(* Logix 5000 AddOnInstructionDefinition export EH_Cerabar_PMP43_IOL; software revision 38.00 *)

TYPE EH_CommAOI_Data :
STRUCT
   Device_Comm_Error : BOOL;
   CommSuccess : BOOL;
   CommFailed : BOOL;
   CommTimeOut : BOOL;
   StateDone : BOOL;
   NewState : BOOL;
   OldState : SINT;
   PortSize : SINT;
   DevicePort : SINT;
   MaxState : SINT;
   State : SINT;
   VendorID : INT;
   DeviceID : DINT;
   CyclicData : INT[16];
   AcyclicData : DINT[8];
   ReplayIndex : INT;
   AOI_Diagnostic : DINT;
   ConnectionStatus : DINT;
   OutputData : INT[16];
END_STRUCT
END_TYPE

ADD_ON_INSTRUCTION EH_Cerabar_PMP43_IOL   (* revision 1.2, vendor Endress+Hauser *)
// Cerabar PMP 43  Rev 1 IO-Link
// Revision note:
// 1.2 Added HeartbeatVerification
// 1.1 Changed the Datatype from Unsigned to Signed
// Add Disconnect check
VAR_IN_OUT
   DataToSend : INT[10]; {required}
   CommAOIBusy : DINT; {required}
   ActiveComPort : DINT; {required}
   DeviceAOISendRequest : DINT; {required}
   CommError : INT; {required}
   DeviceData : EH_CommAOI_Data; {required}
END_VAR
VAR_INPUT
   iSetSimulation : BOOL; {visible}
   iSimulationVariable : INT; {visible}
   iSimulationValue_Pressure : REAL; {visible}
   iSetUnit : BOOL; {visible}
   iUnit : INT; {visible}
   iStart_HeartbeatVerification : BOOL; {visible}
END_VAR
VAR_OUTPUT
   qVendor_ID : DINT; {access Read Only, visible}
   qDevice_ID : DINT; {access Read Only, visible}
   qPressure : REAL; {access None, visible}
   qExtendedDeviceStatus : INT; {access Read Only, visible}
   qUnit : INT; {access Read Only, visible}
   qSSC1_1 : BOOL; {access Read Only, visible}
   qSSC1_2 : BOOL; {access Read Only, visible}
   qVerificationID : INT; {access Read Only, visible}
   qPassed : BOOL; {visible}
   qFailed : BOOL; {visible}
   qAOI_Diagnostic : DINT; {access Read Only, visible}
END_VAR
VAR_IN_OUT
   qAOI_Diagnostic_String : STRING; {required}
END_VAR
VAR_OUTPUT
   qActual_Diagnostics_Code : DINT; {access Read Only, visible}
END_VAR
VAR_IN_OUT
   qActual_Diagnostics_String : STRING; {required}
END_VAR
VAR_OUTPUT
   qLast_Diagnostics_Code : DINT; {visible}
END_VAR
VAR_IN_OUT
   qLast_Diagnostics_String : STRING; {required}
END_VAR
VAR_OUTPUT
   qCommError : DINT; {access None}
   qCommunicationBusy : DINT; {access Read Only, visible}
   qDeviceConnectionError : BOOL; {access Read Only, visible}
END_VAR
VAR
   Temp_DINT : DINT; {access None}
   CMD_Index : INT; {access None}
   CMD_Subindex : INT; {access None}
   CMD_ByteLength : INT; {access None}
   oldCondStatus : INT; {access None}
   oldSetSimulation : SINT; {access None}
   SetSimulation : SINT; {access None}
   SetUnit : SINT; {access None}
   oldSetUnit : SINT; {access None}
   Trigger : BOOL; {access None}
   CMD_Rd : BOOL; {access None}
   CMD_Wr : BOOL; {access None}
   SimulationDINT : DINT; {access None}
   InputByteLength : DINT; {access None}
   AOI_Prio : BOOL; {access None}
   StateMin : DINT; {access None}
   firstTimeDone : BOOL; {access None}
   OldStatus : DINT; {access None}
   CondStatusChanged : BOOL; {access None}
   Calc_ExtendedDeviceStatus : DINT; {access None}
   Totalizer1_DINT : DINT; {access None}
   SimActive : BOOL; {access None}
   CondStatusActive : BOOL; {access None}
   ActiveAOI : BOOL; {access None}
   Skip : BOOL; {access None}
   SimChanged : BOOL; {access None}
   UnitActive : BOOL; {access None}
   UnitChanged : BOOL; {access None}
   DeviceID : DINT; {access None}
   FALSE : BOOL; {access None}
   TRUE : BOOL := 1; {access None}
   temp_string1 : STRING; {access None}
   temp_string2 : STRING; {access None}
   Calc_Pressure : DINT; {access None}
   qPressureTemp : REAL; {access None}
   tempVal : SINT; {access None}
   Start_HeartbeatVerification : SINT; {access None}
   oldStart_HeartbeatVerification : SINT; {access None}
   init : BOOL; {access None}
   SimulationREAL : REAL; {access None}
   StandardTimer : FBD_TIMER; {access None}
   onlyonce : DINT; {access None}
   HeartbeatVerification : BOOL; {access None}
   HeartbeatVerificationActive : BOOL; {access None}
   HeartbeatVerificationChanged : BOOL; {access None}
   b_var : BOOL; {access None}
END_VAR

ROUTINE Logic   (* structured text *)
// Picomag Communication via AL1323
   // =======================================================================
   // Endress+Hauser Digital Solutions
   // ©Copyright (2024) All Rights Reserved
   // =======================================================================
   // Name:                EH_Cerabar_PMP43_IOL
   // Version:             1.2
   // Datum:               11.2025
   // Library:             01.01.00
   // Engineering:         Studio5000 V38.00.00
   // Author:              EH
   // =======================================================================
   
   qAOI_Diagnostic := DeviceData.AOI_Diagnostic;
   qCommunicationBusy := CommAOIBusy;
   DeviceID := 9618689;
   StateMin := 0;
   DeviceData.MaxState := 98;
   
   if DeviceData.DevicePort = 0 or DeviceData.DeviceID <> DeviceID or DeviceData.ConnectionStatus <> 1 then
   
   	qVendor_ID := DeviceData.VendorID;
   	qDevice_ID := DeviceData.DeviceID;
   	qPressure	:= 0;
   	qExtendedDeviceStatus	:= 0;
   	qUnit	:= 0;
   	qSSC1_1	:= FALSE;
   	qSSC1_2	:= FALSE;
   	qActual_Diagnostics_Code	:= 0;
   	qLast_Diagnostics_Code	:= 0;
   	qLast_Diagnostics_String	:= '';
   	qVendor_ID := 0;
   	qPassed := FALSE;
   	qFailed := FALSE;
   	oldCondStatus := 0;
   	CondStatusChanged := FALSE;
   	init := FALSE;
   
   	if DeviceData.DevicePort = 0 then
   
   		qActual_Diagnostics_String	:= 'Device Port is Zero';
   		DeviceData.AOI_Diagnostic.1 := TRUE;
   
   	elsif DeviceData.ConnectionStatus <> 1 then
   
   		qActual_Diagnostics_String	:= 'No Device connected';
   		qDeviceConnectionError := TRUE;
   
   	elsif DeviceData.DeviceID <> DeviceID then
   
   		qActual_Diagnostics_String	:= 'Wrong DeviceID';
   		DeviceData.AOI_Diagnostic.2 := TRUE;
   
   	end_if;
   
   else
   
   	if qActual_Diagnostics_Code = 0  then
   
   		qActual_Diagnostics_String	:= '--------';
   
   	end_if;
   
   	if qLast_Diagnostics_Code = 0 then
   
   		qLast_Diagnostics_String	:= '--------';
   
   	end_if;
   
   	DeviceData.AOI_Diagnostic.1 := FALSE;
   	qDeviceConnectionError := FALSE;
   	DeviceData.AOI_Diagnostic.2  := FALSE;
   
   end_if;
   
   if not DeviceData.AOI_Diagnostic.0
   	and not qDeviceConnectionError
   	and not DeviceData.AOI_Diagnostic.2
   	and DeviceData.DevicePort > 0 or ActiveAOI and qDeviceConnectionError then
   
   	//*********************************
   	//Vendor ID
   	//*********************************
   
   		qVendor_ID := DeviceData.VendorID;
   
   	//*********************************
   	//Device ID
   	//*********************************
   
   		qDevice_ID := DeviceData.DeviceID;
   
   	//*********************************
   	// PMP43
   	//*********************************
   
   		Calc_Pressure				:= 0;
   		Calc_ExtendedDeviceStatus	:= 2;
   
   	//*********************************
   	//Process Data Pressure
   	//*********************************
   
   		Temp_DINT	 := DeviceData.CyclicData[Calc_Pressure+1];
   		Temp_DINT.8	 := DeviceData.CyclicData[Calc_Pressure+1].8;
   		Temp_DINT.9  := DeviceData.CyclicData[Calc_Pressure+1].9;
   		Temp_DINT.10 := DeviceData.CyclicData[Calc_Pressure+1].10;
   		Temp_DINT.11 := DeviceData.CyclicData[Calc_Pressure+1].11;
   		Temp_DINT.12 := DeviceData.CyclicData[Calc_Pressure+1].12;
   		Temp_DINT.13 := DeviceData.CyclicData[Calc_Pressure+1].13;
   		Temp_DINT.14 := DeviceData.CyclicData[Calc_Pressure+1].14;
   		Temp_DINT.15 := DeviceData.CyclicData[Calc_Pressure+1].15;
   		Temp_DINT.16 := DeviceData.CyclicData[Calc_Pressure].0;
   		Temp_DINT.17 := DeviceData.CyclicData[Calc_Pressure].1;
   		Temp_DINT.18 := DeviceData.CyclicData[Calc_Pressure].2;
   		Temp_DINT.19 := DeviceData.CyclicData[Calc_Pressure].3;
   		Temp_DINT.20 := DeviceData.CyclicData[Calc_Pressure].4;
   		Temp_DINT.21 := DeviceData.CyclicData[Calc_Pressure].5;
   		Temp_DINT.22 := DeviceData.CyclicData[Calc_Pressure].6;
   		Temp_DINT.23 := DeviceData.CyclicData[Calc_Pressure].7;
   		Temp_DINT.24 := DeviceData.CyclicData[Calc_Pressure].8;
   		Temp_DINT.25 := DeviceData.CyclicData[Calc_Pressure].9;
   		Temp_DINT.26 := DeviceData.CyclicData[Calc_Pressure].10;
   		Temp_DINT.27 := DeviceData.CyclicData[Calc_Pressure].11;
   		Temp_DINT.28 := DeviceData.CyclicData[Calc_Pressure].12;
   		Temp_DINT.29 := DeviceData.CyclicData[Calc_Pressure].13;
   		Temp_DINT.30 := DeviceData.CyclicData[Calc_Pressure].14;
   		Temp_DINT.31 := DeviceData.CyclicData[Calc_Pressure].15;
   
   		case qUnit of
   
   			//*********************************
   			0: // bar
   			//*********************************
   			COP(Temp_DINT,qPressureTemp,1);
   			qPressure := qPressureTemp / 100000;
   
   			//*********************************
   			6: // psi
   			//*********************************
   			COP(Temp_DINT,qPressureTemp,1);
   			qPressure := qPressureTemp / 6895.7573;
   
   			//*********************************
   			8: // mbar
   			//*********************************
   			COP(Temp_DINT,qPressureTemp,1);
   			qPressure := qPressureTemp / 100;
   
   			//*********************************
   			11: // Pa
   			//*********************************
   			COP(Temp_DINT,qPressure,1);
   
   			//*********************************
   			12: // kPa
   			//*********************************
   			COP(Temp_DINT,qPressureTemp,1);
   			qPressure := qPressureTemp / 1000;
   
   			//*********************************
   			237: // MPA
   			//*********************************
   			COP(Temp_DINT,qPressureTemp,1);
   			qPressure := qPressureTemp / 1000000;
   
   			else // Base unit, Pa
   				COP(Temp_DINT,qPressure,1);
   
   		end_case;
   
   	//*********************************
   	// Extended device Status
   	//*********************************
   
   		qExtendedDeviceStatus.0 := DeviceData.CyclicData[Calc_ExtendedDeviceStatus].8;
   		qExtendedDeviceStatus.1 := DeviceData.CyclicData[Calc_ExtendedDeviceStatus].9;
   		qExtendedDeviceStatus.2 := DeviceData.CyclicData[Calc_ExtendedDeviceStatus].10;
   		qExtendedDeviceStatus.3 := DeviceData.CyclicData[Calc_ExtendedDeviceStatus].11;
   		qExtendedDeviceStatus.4 := DeviceData.CyclicData[Calc_ExtendedDeviceStatus].12;
   		qExtendedDeviceStatus.5 := DeviceData.CyclicData[Calc_ExtendedDeviceStatus].13;
   		qExtendedDeviceStatus.6 := DeviceData.CyclicData[Calc_ExtendedDeviceStatus].14;
   		qExtendedDeviceStatus.7 := DeviceData.CyclicData[Calc_ExtendedDeviceStatus].15;
   
   	//*********************************
   	// Process Parameter SSC
   	//*********************************
   
   		qSSC1_1 := DeviceData.CyclicData[Calc_ExtendedDeviceStatus].0;
   		qSSC1_2 := DeviceData.CyclicData[Calc_ExtendedDeviceStatus].1;
   
   	//*********************************
   	// Checking for Changed Status
   	//*********************************
   
   		SetSimulation.0 := iSetSimulation;
   		SetUnit.0 := iSetUnit;
   		Start_HeartbeatVerification.0 := iStart_HeartbeatVerification;
   
   	if oldCondStatus <> qExtendedDeviceStatus and not CondStatusChanged then
   
   		CondStatusChanged := TRUE;
   		oldCondStatus := qExtendedDeviceStatus;
   
   	end_if;
   
   	if oldSetSimulation <> SetSimulation and not SimChanged then
   
   		if oldSetSimulation < SetSimulation then
   
   			SimChanged := TRUE;
   
   		end_if;
   
   		oldSetSimulation := SetSimulation;
   
   	end_if;
   
   	if oldSetUnit <> SetUnit and not UnitChanged then
   
   		if oldSetUnit < SetUnit then
   
   			UnitChanged := TRUE;
   
   		end_if;
   
   		oldSetUnit := SetUnit;
   
   	end_if;
   
   	if oldStart_HeartbeatVerification <> Start_HeartbeatVerification and not HeartbeatVerificationChanged then
   
   		if oldStart_HeartbeatVerification < Start_HeartbeatVerification then
   
   			HeartbeatVerificationChanged := TRUE;
   
   		end_if;
   
   		oldStart_HeartbeatVerification := Start_HeartbeatVerification;
   
   	end_if;
   
   	if CondStatusChanged
   		and not ActiveAOI
   		and not CondStatusActive
   		and not Skip then
   
   		DeviceAOISendRequest.[DeviceData.DevicePort] := TRUE;
   		CondStatusActive := TRUE;
   		Skip := TRUE;
   
   	elsif SimChanged
   		and not ActiveAOI
   		and not SimActive
   		and not Skip then
   
   		DeviceAOISendRequest.[DeviceData.DevicePort] := TRUE;
   		SimActive := TRUE;
   		Skip := TRUE;
   
   	elsif UnitChanged
   		and not ActiveAOI
   		and not UnitActive
   		and not Skip then
   
   		DeviceAOISendRequest.[DeviceData.DevicePort] := TRUE;
   		UnitActive := TRUE;
   		Skip := TRUE;
   
   	elsif HeartbeatVerificationChanged
   		and not ActiveAOI
   		and not HeartbeatVerificationActive
   		and not Skip then
   
   		DeviceAOISendRequest.[DeviceData.DevicePort] := TRUE;
   		HeartbeatVerificationActive := TRUE;
   		Skip := TRUE;
   
   	end_if;
   
   end_if;
   
   	if ActiveComPort = DeviceData.DevicePort then
   
   		AOI_Prio := TRUE;
   
   	else
   
   		AOI_Prio := FALSE;
   
   	end_if;
   
   	if (SimActive or UnitActive or HeartbeatVerificationActive or CondStatusActive ) and CommAOIBusy = 1  and DeviceData.State = 0 and AOI_Prio and not ActiveAOI then
   
   		ActiveAOI := TRUE;
   		Skip := FALSE;
   
   	end_if;
   
   	qCommunicationBusy := CommAOIBusy;
   	qAOI_Diagnostic :=DeviceData.AOI_Diagnostic;
   
   	//*********************************
   	// States for Execution
   	//*********************************
   
   	if ActiveAOI or DeviceData.State = DeviceData.MaxState then
   
   	case DeviceData.State of
   
   		//*********************************
   		0: // Idle
   		//*********************************
   
   			// Initializing
   			Trigger := 0;
   			CMD_Index := 0;
   			CMD_Subindex := 0;
   			CMD_Wr := FALSE;
   			CMD_Rd := FALSE;
   		    CMD_ByteLength := 0;
   
   			if DeviceData.DevicePort = ActiveComPort then
   
   					DeviceData.CommSuccess := FALSE;
   					DeviceData.CommTimeOut := FALSE;
   					DeviceData.NewState := TRUE;
   					DeviceData.StateDone := FALSE;
   
   			end_if;
   
   			// Wait for trigger
   			if SimActive then
   
   				DeviceData.AOI_Diagnostic := 0;
   				DeviceData.State := 1;
   
   			elsif UnitActive then
   
   				DeviceData.AOI_Diagnostic := 0;
   				DeviceData.State := 4;
   
   			elsif HeartbeatVerificationActive then
   
   				DeviceData.AOI_Diagnostic := 0;
   				DeviceData.State := 80;
   
   			elsif CondStatusChanged then
   
   				if not init then
   
   					DeviceData.State := 5;
   
   				else
   
   					DeviceData.State := 90;
   
   				end_if;
   
   			end_if;
   
   
   	//*********************************
   	1: // Set Simulation Variable
   	//*********************************
   
   			CMD_Index := 1332;
   			CMD_Subindex := 0;
   			CMD_Wr := TRUE;								// Only Read or Write can be active = 1
   			CMD_Rd := FALSE;
   			CMD_ByteLength := 2;
   			DataToSend[6]:= 0;
   			DataToSend[7]:= 0;
   
   			if iSimulationVariable > 0 then
   				tempVal := 22;
   				DataToSend[6] := 0;
   				DataToSend[6].8 := tempVal.0;
   				DataToSend[6].9 := tempVal.1;
   				DataToSend[6].10 := tempVal.2;
   				DataToSend[6].11 := tempVal.3;
   				DataToSend[6].12 := tempVal.4;
   				DataToSend[6].13 := tempVal.5;
   				DataToSend[6].14 := tempVal.6;
   				DataToSend[6].15 := tempVal.7;
   
   			else
   				DataToSend[6] := 0;
   				DataToSend[7] := 0;
   			end_if;
   
   			Trigger := TRUE;
   
   			if DeviceData.NewState then
   				DeviceData.StateDone := TRUE;
   			end_if;
   
   			if  DeviceData.CommSuccess and DeviceData.ReplayIndex = CMD_Index then
   
   				Trigger := FALSE;
   				DeviceData.OldState := DeviceData.State;
   				DeviceData.State := DeviceData.State + 1;
   				DeviceData.CommSuccess := FALSE;
   				DeviceData.AcyclicData[0] := 0;
   				DeviceData.NewState := TRUE;
   			elsif DeviceData.CommTimeOut then
   
   				temp_string1 := 'Error in step ';
   				Temp_DINT := DeviceData.State;
   				DTOS(Temp_DINT, temp_string2);
   				CONCAT(temp_string1, temp_string2, qAOI_Diagnostic_String);
   
   				DeviceData.OldState := DeviceData.State;
   				DeviceData.State := DeviceData.MaxState;
   				DeviceData.CommTimeOut := FALSE;
   				DeviceData.AcyclicData[0] := 0;
   				DeviceData.NewState := TRUE;
   			end_if;
   
   		//*********************************
   		2: // Set Simulation Value
   		//*********************************
   
   			CMD_Index := 8542;
   			CMD_Subindex := 0;
   			CMD_Wr := TRUE;								// Only Read or Write can be active = 1
   			CMD_Rd := FALSE;
   			CMD_ByteLength := 4;
   			DataToSend[6]:= 0;
   			DataToSend[7]:= 0;
   
   			case qUnit of
   
   			//*********************************
   			0: // bar
   			//*********************************
   			SimulationREAL := iSimulationValue_Pressure * 100000;
   
   			//*********************************
   			6: // psi
   			//*********************************
   			SimulationREAL := iSimulationValue_Pressure * 6895.7573;
   
   			//*********************************
   			8: // mbar
   			//*********************************
   			SimulationREAL := iSimulationValue_Pressure * 100;
   
   			//*********************************
   			11: // Pa
   			//*********************************
   			SimulationREAL := iSimulationValue_Pressure;
   
   			//*********************************
   			12: // kPa
   			//*********************************
   			SimulationREAL := iSimulationValue_Pressure * 1000;
   
   			//*********************************
   			237: // MPA
   			//*********************************
   			SimulationREAL := iSimulationValue_Pressure * 1000000;
   
   			else // Base unit, Pa
   				SimulationREAL := iSimulationValue_Pressure;
   
   		end_case;
   
   		 	COP(SimulationREAL,SimulationDINT,1); // Copy the Bits from the Real in a DINT
   
   			DataToSend[6].0 :=  SimulationDINT.24;
   			DataToSend[6].1 :=  SimulationDINT.25;
   			DataToSend[6].2 :=  SimulationDINT.26;
   			DataToSend[6].3 :=  SimulationDINT.27;
   			DataToSend[6].4 :=  SimulationDINT.28;
   			DataToSend[6].5 :=  SimulationDINT.29;
   			DataToSend[6].6 :=  SimulationDINT.30;
   			DataToSend[6].7 :=  SimulationDINT.31;
   			DataToSend[6].8 :=  SimulationDINT.16;
   			DataToSend[6].9 :=  SimulationDINT.17;
   			DataToSend[6].10 := SimulationDINT.18;
   			DataToSend[6].11 := SimulationDINT.19;
   			DataToSend[6].12 := SimulationDINT.20;
   			DataToSend[6].13 := SimulationDINT.21;
   			DataToSend[6].14 := SimulationDINT.22;
   			DataToSend[6].15 := SimulationDINT.23;
   			DataToSend[7].0  := SimulationDINT.8;
   			DataToSend[7].1  := SimulationDINT.9;
   			DataToSend[7].2  := SimulationDINT.10;
   			DataToSend[7].3  := SimulationDINT.11;
   			DataToSend[7].4  := SimulationDINT.12;
   			DataToSend[7].5  := SimulationDINT.13;
   			DataToSend[7].6  := SimulationDINT.14;
   			DataToSend[7].7  := SimulationDINT.15;
   			DataToSend[7].8  := SimulationDINT.0;
   			DataToSend[7].9  := SimulationDINT.1;
   			DataToSend[7].10 := SimulationDINT.2;
   			DataToSend[7].11 := SimulationDINT.3;
   			DataToSend[7].12 := SimulationDINT.4;
   			DataToSend[7].13 := SimulationDINT.5;
   			DataToSend[7].14 := SimulationDINT.6;
   			DataToSend[7].15 := SimulationDINT.7;
   
   			Trigger := TRUE;
   
   			if DeviceData.NewState then
   				DeviceData.StateDone := TRUE;
   			end_if;
   
   			if  DeviceData.CommSuccess and DeviceData.ReplayIndex = CMD_Index then
   
   				Trigger := FALSE;
   				DeviceData.OldState := DeviceData.State;
   				DeviceData.State := DeviceData.MaxState;
   				DeviceData.CommSuccess := FALSE;
   				DeviceData.AcyclicData[0] := 0;
   				DeviceData.NewState := TRUE;
   
   		 	elsif DeviceData.CommTimeOut then
   
   				temp_string1 := 'Error in step ';
   				Temp_DINT := DeviceData.State;
   				DTOS(Temp_DINT, temp_string2);
   				CONCAT(temp_string1, temp_string2, qAOI_Diagnostic_String);
   
   				DeviceData.OldState := DeviceData.State;
   				DeviceData.State := DeviceData.MaxState;
   				DeviceData.CommTimeOut := FALSE;
   				DeviceData.AcyclicData[0] := 0;
   				DeviceData.NewState := TRUE;
   
   			end_if;
   
   		//*********************************
   		4: // Set unit
   		//*********************************
   
   			CMD_Index := 316;
   			CMD_Subindex := 0;
   			CMD_Wr := TRUE;								// Only Read or Write can be active = 1
   			CMD_Rd := FALSE;
   			CMD_ByteLength := 2;
   			DataToSend[6] := 0;
   			DataToSend[7] := 0;
   
   			if iUnit = 0 OR iUnit = 6 OR iUnit = 8 OR iUnit = 11 OR iUnit = 12 OR iUnit = 237 then
   
   				DataToSend[6].8 := iUnit.0;
   				DataToSend[6].9 := iUnit.1;
   				DataToSend[6].10 := iUnit.2;
   				DataToSend[6].11 := iUnit.3;
   				DataToSend[6].12 := iUnit.4;
   				DataToSend[6].13 := iUnit.5;
   				DataToSend[6].14 := iUnit.6;
   				DataToSend[6].15 := iUnit.7;
   
   				Trigger := TRUE;
   
   				if DeviceData.NewState then
   
   					DeviceData.StateDone := TRUE;
   
   				end_if;
   
   				if  DeviceData.CommSuccess and DeviceData.ReplayIndex = CMD_Index then
   
   					Trigger := FALSE;
   					DeviceData.OldState := DeviceData.State;
   					DeviceData.State := DeviceData.State + 1;
   					DeviceData.CommSuccess := FALSE;
   					DeviceData.AcyclicData[0] := 0;
   					DeviceData.NewState := TRUE;
   
   			 	elsif DeviceData.CommTimeOut then
   
   					temp_string1 := 'Error in step ';
   					Temp_DINT := DeviceData.State;
   					DTOS(Temp_DINT, temp_string2);
   					CONCAT(temp_string1, temp_string2, qAOI_Diagnostic_String);
   
   					DeviceData.OldState := DeviceData.State;
   					DeviceData.State := DeviceData.MaxState;	//Check State
   					DeviceData.CommTimeOut := FALSE;
   					DeviceData.AcyclicData[0] := 0;
   					DeviceData.NewState := TRUE;
   
   				end_if;
   
   			else
   
   					temp_string1 := 'Error in step ';
   					Temp_DINT := DeviceData.State;
   					DTOS(Temp_DINT, temp_string2);
   					CONCAT(temp_string1, temp_string2, qAOI_Diagnostic_String);
   
   					DeviceData.OldState := DeviceData.State;
   					DeviceData.State := DeviceData.MaxState;
   					DeviceData.CommTimeOut := FALSE;
   					DeviceData.AcyclicData[0] := 0;
   					DeviceData.NewState := TRUE;
   
   	        end_if;
   
   
   		//*********************************
   		5: // Read Unit
   		//*********************************
   
   			CMD_Index := 316;
   			CMD_Subindex := 0;
   			CMD_Wr := FALSE;
   			CMD_Rd := TRUE;
   			CMD_ByteLength := 2;
   			Trigger := TRUE;
   
   			if DeviceData.NewState then
   				DeviceData.StateDone := TRUE;
   			end_if;
   
   			if  DeviceData.CommSuccess and DeviceData.ReplayIndex = CMD_Index then
   
   				qUnit.0	:= DeviceData.AcyclicData[0].0;
   				qUnit.1	:= DeviceData.AcyclicData[0].1;
   				qUnit.2	:= DeviceData.AcyclicData[0].2;
   				qUnit.3	:= DeviceData.AcyclicData[0].3;
   				qUnit.4	:= DeviceData.AcyclicData[0].4;
   				qUnit.5	:= DeviceData.AcyclicData[0].5;
   				qUnit.6	:= DeviceData.AcyclicData[0].6;
   				qUnit.7	:= DeviceData.AcyclicData[0].7;
   
   				Trigger := FALSE;
   
   				DeviceData.OldState := DeviceData.State;
   				DeviceData.State := DeviceData.MaxState;
   				DeviceData.CommSuccess := FALSE;
   				DeviceData.AcyclicData[0] := 0;
   				DeviceData.NewState := TRUE;
   
   				if not init then
   
   					init := TRUE;
   					DeviceData.State := 90;
   
   				end_if;
   
   			 elsif DeviceData.CommTimeOut then
   
   				temp_string1 := 'Error in step ';
   				Temp_DINT := DeviceData.State;
   				DTOS(Temp_DINT, temp_string2);
   				CONCAT(temp_string1, temp_string2, qAOI_Diagnostic_String);
   
   				DeviceData.OldState := DeviceData.State;
   				DeviceData.State := DeviceData.MaxState;
   				DeviceData.CommTimeOut := FALSE;
   				DeviceData.AcyclicData[0] := 0;
   				DeviceData.NewState := TRUE;
   
   			end_if;
   
   		//*********************************
   		80: // Check Heartbeat Verification activation
   		//*********************************
   
   			CMD_Index := 12342;
   			CMD_Subindex := 0;
   			CMD_Wr := FALSE;
   			CMD_Rd := TRUE;
   			CMD_ByteLength := 1;
   			Trigger := TRUE;
   			DataToSend[6]:= 0;
   			DataToSend[7]:= 0;
   
   			if DeviceData.NewState then
   
   				DeviceData.StateDone := TRUE;
   
   			end_if;
   
   			if  DeviceData.CommSuccess and DeviceData.ReplayIndex = CMD_Index then
   
   				if DeviceData.AcyclicData[0] = 1 then
   
   					DeviceData.State := DeviceData.State + 1;
   
   				else
   					qAOI_Diagnostic_String := 'Step 80: Software Option not activated ';
   
   					DeviceData.OldState := DeviceData.State;
   					DeviceData.State := DeviceData.MaxState;
   
   				end_if;
   
   				Trigger := FALSE;
   				DeviceData.CommSuccess := FALSE;
   				DeviceData.AcyclicData[0] := 0;
   				DeviceData.NewState := TRUE;
   
   			 elsif DeviceData.CommTimeOut then
   
   				temp_string1 := 'Error in step ';
   				Temp_DINT := DeviceData.State;
   				DTOS(Temp_DINT, temp_string2);
   				CONCAT(temp_string1, temp_string2, qAOI_Diagnostic_String);
   
   				DeviceData.OldState := DeviceData.State;
   				DeviceData.State := DeviceData.MaxState;
   				DeviceData.CommTimeOut := FALSE;
   				DeviceData.AcyclicData[0] := 0;
   				DeviceData.NewState := TRUE;
   
   			end_if;
   
   		//*********************************
   		81: // Check if Verifivation is ongoing
   		//*********************************
   
   			CMD_Index := 12323;
   			CMD_Subindex := 0;
   			CMD_Wr := FALSE;
   			CMD_Rd := TRUE;
   			CMD_ByteLength := 2;
   			Trigger := TRUE;
   
   			if DeviceData.NewState then
   
   				DeviceData.StateDone := TRUE;
   
   			end_if;
   
   			if  DeviceData.CommSuccess and DeviceData.ReplayIndex = CMD_Index then
   
   				if DeviceData.AcyclicData[0] <> 8 then
   
   					DeviceData.State := DeviceData.State + 1;
   
   				else
   					qAOI_Diagnostic_String := 'Step 81: Heartbeat Verification already in progress ';
   					DeviceData.OldState := DeviceData.State;
   					DeviceData.State := DeviceData.MaxState;
   					DeviceData.CommTimeOut := FALSE;
   
   				end_if;
   
   				Trigger := FALSE;
   				DeviceData.CommSuccess := FALSE;
   				DeviceData.AcyclicData[0] := 0;
   				DeviceData.NewState := TRUE;
   
   			 elsif DeviceData.CommTimeOut then
   
   				temp_string1 := 'Error in step ';
   				Temp_DINT := DeviceData.State;
   				DTOS(Temp_DINT, temp_string2);
   				CONCAT(temp_string1, temp_string2, qAOI_Diagnostic_String);
   
   				DeviceData.OldState := DeviceData.State;
   				DeviceData.State := DeviceData.MaxState;
   				DeviceData.CommTimeOut := FALSE;
   				DeviceData.AcyclicData[0] := 0;
   				DeviceData.NewState := TRUE;
   
   			end_if;
   
   		//*********************************
   		82: // Start Verification
   		//*********************************
   
   			CMD_Index := 12325;
   			CMD_Subindex := 0;
   			CMD_Wr := TRUE;
   			CMD_Rd := FALSE;
   			CMD_ByteLength := 2;
   			Trigger := TRUE;
   			DataToSend[6] := 0;
   			DataToSend[7] := 0;
   
   			DataToSend[6].8 := TRUE;
   
   			if DeviceData.NewState then
   
   				DeviceData.StateDone := TRUE;
   
   			end_if;
   
   		if DeviceData.CommSuccess and DeviceData.ReplayIndex = CMD_Index then
   
   		    Trigger := FALSE;
   		    DeviceData.CommSuccess := FALSE;
   		    DeviceData.State := DeviceData.State + 3;
   			DeviceData.AcyclicData[0] := 0;
   			DeviceData.NewState := TRUE;
   
   		elsif DeviceData.CommTimeOut then
   
   		    temp_string1 := 'Error in step ';
   		    Temp_DINT := DeviceData.State;
   		    DTOS(Temp_DINT, temp_string2);
   		    CONCAT(temp_string1, temp_string2, qAOI_Diagnostic_String);
   
   		    DeviceData.OldState := DeviceData.State;
   		    DeviceData.State := DeviceData.MaxState;
   		    DeviceData.CommTimeOut := FALSE;
   			DeviceData.AcyclicData[0] := 0;
   			DeviceData.NewState := TRUE;
   
   		end_if;
   
   
   		//*********************************
   		83: // Intermediate state
   		//*********************************
   
   			CMD_Index := 36;
   			CMD_Subindex := 0;
   			CMD_Wr := FALSE;
   			CMD_Rd := TRUE;
   			CMD_ByteLength := 1;
   			Trigger := TRUE;
   
   			if DeviceData.NewState then
   
   				DeviceData.StateDone := TRUE;
   
   			end_if;
   
   			if DeviceData.CommSuccess and DeviceData.ReplayIndex = CMD_Index then
   
   			    DeviceData.State := DeviceData.State + 2;
   			    Trigger := FALSE;
   			    DeviceData.CommSuccess := FALSE;
   				DeviceData.AcyclicData[0] := 0;
   				DeviceData.NewState := TRUE;
   
   			elsif DeviceData.CommTimeOut then
   
   			    temp_string1 := 'Error in step ';
   			    Temp_DINT := DeviceData.State;
   			    DTOS(Temp_DINT, temp_string2);
   			    CONCAT(temp_string1, temp_string2, qAOI_Diagnostic_String);
   
   			    DeviceData.OldState := DeviceData.State;
   			    DeviceData.State := DeviceData.MaxState;
   			    DeviceData.CommTimeOut := FALSE;
   				DeviceData.AcyclicData[0] := 0;
   				DeviceData.NewState := TRUE;
   
   			end_if;
   
   		//*********************************
   		84: // Read progress
   		//*********************************
   
   		//*********************************
   		85: // Read status
   		//*********************************
   
   			CMD_Index := 12323;
   			CMD_Subindex := 0;
   			CMD_Wr := FALSE;
   			CMD_Rd := TRUE;
   			CMD_ByteLength := 2;
   			Trigger := TRUE;
   
   			if DeviceData.NewState then
   
   				DeviceData.StateDone := TRUE;
   
   			end_if;
   
   			if DeviceData.CommSuccess and DeviceData.ReplayIndex = CMD_Index then
   
   			    if DeviceData.AcyclicData[0] = 10 then
   
   			        DeviceData.State := DeviceData.State + 1;
   
   			    elsif DeviceData.AcyclicData[0] = 8 then
   
   					DeviceData.State := DeviceData.State - 2;
   
   			    else
   			        qAOI_Diagnostic_String := 'Step 85: Heartbeat Verification not done';
   			        DeviceData.OldState := DeviceData.State;
   			        DeviceData.State := DeviceData.MaxState;
   			        DeviceData.CommTimeOut := FALSE;
   
   			    end_if;
   
   			    Trigger := FALSE;
   			    DeviceData.CommSuccess := FALSE;
   				DeviceData.AcyclicData[0] := 0;
   				DeviceData.NewState := TRUE;
   
   			elsif DeviceData.CommTimeOut then
   
   			    temp_string1 := 'Error in step ';
   			    Temp_DINT := DeviceData.State;
   			    DTOS(Temp_DINT, temp_string2);
   			    CONCAT(temp_string1, temp_string2, qAOI_Diagnostic_String);
   
   			    DeviceData.OldState := DeviceData.State;
   			    DeviceData.State := DeviceData.MaxState;
   			    DeviceData.CommTimeOut := FALSE;
   				DeviceData.AcyclicData[0] := 0;
   				DeviceData.NewState := TRUE;
   
   			end_if;
   
   		//*********************************
   		86: // Read overall result
   		//*********************************
   
   			CMD_Index := 1396;
   			CMD_Subindex := 0;
   			CMD_Wr := FALSE;
   			CMD_Rd := TRUE;
   			CMD_ByteLength := 2;
   			Trigger := TRUE;
   
   			if DeviceData.NewState then
   
   				DeviceData.StateDone := TRUE;
   
   			end_if;
   
   			if  DeviceData.CommSuccess and DeviceData.ReplayIndex = CMD_Index then
   
   				if DeviceData.AcyclicData[0] = 1 then
   
   					qPassed := TRUE;
   					qFailed := FALSE;
   
   				else
   
   					qPassed := FALSE;
   					qFailed := TRUE;
   
   				end_if;
   
   				Trigger := FALSE;
   				DeviceData.CommSuccess := FALSE;
   				DeviceData.State := DeviceData.State + 1;
   				DeviceData.AcyclicData[0] := 0;
   				DeviceData.NewState := TRUE;
   
   			 elsif DeviceData.CommTimeOut then
   
   				temp_string1 := 'Error in step ';
   				Temp_DINT := DeviceData.State;
   				DTOS(Temp_DINT, temp_string2);
   				CONCAT(temp_string1, temp_string2, qAOI_Diagnostic_String);
   
   				DeviceData.CommTimeOut := FALSE;
   				DeviceData.OldState := DeviceData.State;
   				DeviceData.State := DeviceData.MaxState;
   				DeviceData.AcyclicData[0] := 0;
   				DeviceData.NewState := TRUE;
   
   			end_if;
   
   		//*********************************
   		87: // Read Verification ID
   		//*********************************
   
   			CMD_Index := 12321;
   			CMD_Subindex := 0;
   			CMD_Wr := FALSE;
   			CMD_Rd := TRUE;
   			CMD_ByteLength := 2;
   			Trigger := TRUE;
   
   			if DeviceData.NewState then
   
   				DeviceData.StateDone := TRUE;
   
   			end_if;
   
   			if  DeviceData.CommSuccess and DeviceData.ReplayIndex = CMD_Index then
   
   				qVerificationID.0	:= DeviceData.AcyclicData[0].0;
   				qVerificationID.1	:= DeviceData.AcyclicData[0].1;
   				qVerificationID.2	:= DeviceData.AcyclicData[0].2;
   				qVerificationID.3	:= DeviceData.AcyclicData[0].3;
   				qVerificationID.4	:= DeviceData.AcyclicData[0].4;
   				qVerificationID.5	:= DeviceData.AcyclicData[0].5;
   				qVerificationID.6	:= DeviceData.AcyclicData[0].6;
   				qVerificationID.7	:= DeviceData.AcyclicData[0].7;
   				qVerificationID.8	:= DeviceData.AcyclicData[0].8;
   				qVerificationID.9	:= DeviceData.AcyclicData[0].9;
   				qVerificationID.10	:= DeviceData.AcyclicData[0].10;
   				qVerificationID.11	:= DeviceData.AcyclicData[0].11;
   				qVerificationID.12	:= DeviceData.AcyclicData[0].12;
   				qVerificationID.13	:= DeviceData.AcyclicData[0].13;
   				qVerificationID.14	:= DeviceData.AcyclicData[0].14;
   				qVerificationID.15	:= DeviceData.AcyclicData[0].15;
   
   				Trigger := FALSE;
   				DeviceData.CommSuccess := FALSE;
   				DeviceData.OldState := DeviceData.State;
   				DeviceData.State := DeviceData.MaxState;
   				DeviceData.NewState := TRUE;
   
   			 elsif DeviceData.CommTimeOut then
   
   				temp_string1 := 'Error in step ';
   				Temp_DINT := DeviceData.State;
   				DTOS(Temp_DINT, temp_string2);
   				CONCAT(temp_string1, temp_string2, qAOI_Diagnostic_String);
   
   				DeviceData.CommTimeOut := FALSE;
   				DeviceData.OldState := DeviceData.State;
   				DeviceData.State := DeviceData.MaxState;
   				DeviceData.NewState := TRUE;
   
   			end_if;
   
   		//*********************************
   		90: // Actual Diagnostic
   		//*********************************
   
   			CMD_Index := 297;
   			CMD_Subindex := 0;
   			CMD_Wr := FALSE;
   			CMD_Rd := TRUE;
   			CMD_ByteLength := 4;
   			Trigger := TRUE;
   
   			if DeviceData.NewState then
   				DeviceData.StateDone := 1;
   			end_if;
   
   			if  DeviceData.CommSuccess and DeviceData.ReplayIndex = CMD_Index then
   
   				qActual_Diagnostics_Code	:= DeviceData.AcyclicData[0];
   
   				case qActual_Diagnostics_Code of
   
   				0:
   		            qActual_Diagnostics_String := '--------';
   		        16777241:
   		            qActual_Diagnostics_String := 'F841 Operating range';
   		        16777245:
   		            qActual_Diagnostics_String := 'F081 Sensor initialization faulty';
   		        16777246:
   		            qActual_Diagnostics_String := 'F100 Sensor error';
   		        16777250:
   		            qActual_Diagnostics_String := 'F062 Sensor connection faulty';
   		        16777253:
   		            qActual_Diagnostics_String := 'F822 Sensor temperature out of range';
   		        16777259:
   		            qActual_Diagnostics_String := 'F801 Supply voltage too low';
   		        16777267:
   		            qActual_Diagnostics_String := 'F435 Linearization faulty';
   		        16777283:
   		            qActual_Diagnostics_String := 'F803 Loop current faulty';
   		        16777297:
   		            qActual_Diagnostics_String := 'F102 Sensor incompatible error';
   		        16777312:
   		            qActual_Diagnostics_String := 'F437 Configuration incompatible';
   		        16777314:
   		            qActual_Diagnostics_String := 'F282 Data storage inconsistent';
   		        16777319:
   		            qActual_Diagnostics_String := 'F242 Firmware incompatible';
   		        16777323:
   		            qActual_Diagnostics_String := 'F252 Module incompatible';
   		        16777336:
   		            qActual_Diagnostics_String := 'F270 Main electronics defective';
   		        16777337:
   		            qActual_Diagnostics_String := 'F272 Main electronics faulty';
   		        16777340:
   		            qActual_Diagnostics_String := 'F270 Main electronics defective';
   		        16777341:
   		            qActual_Diagnostics_String := 'F272 Main electronics faulty';
   		        16777343:
   		            qActual_Diagnostics_String := 'F270 Main electronics defective';
   		        16777344:
   		            qActual_Diagnostics_String := 'F270 Main electronics defective';
   		        16777348:
   		            qActual_Diagnostics_String := 'F270 Main electronics defective';
   		        16777355:
   		            qActual_Diagnostics_String := 'F410 Data transfer failed';
   		        16777374:
   		            qActual_Diagnostics_String := 'F283 Memory content inconsistent';
   		        16777375:
   		            qActual_Diagnostics_String := 'F270 Main electronics defective';
   		        16777387:
   		            qActual_Diagnostics_String := 'F270 Main electronics defective';
   		        16777389:
   		            qActual_Diagnostics_String := 'F805 Loop current faulty';
   		        16777441:
   		            qActual_Diagnostics_String := 'F283 Memory content inconsistent';
   		        16777445:
   		            qActual_Diagnostics_String := 'F273 Main electronics defective';
   		        16777446:
   		            qActual_Diagnostics_String := 'F388 Electronics and HistoROM defective';
   		        16777816:
   		            qActual_Diagnostics_String := 'F272 Main electronics faulty';
   		        16778201:
   		            qActual_Diagnostics_String := 'F501 Process alert scaled variable';
   		        16778202:
   		            qActual_Diagnostics_String := 'F906 Out of range signal detected';
   		        16778203:
   		            qActual_Diagnostics_String := 'F500 Process alert pressure';
   		        16778204:
   		            qActual_Diagnostics_String := 'F502 Process alert temperature';
   		        16778237:
   		            qActual_Diagnostics_String := 'F901 Low signal noise detected';
   		        16778238:
   		            qActual_Diagnostics_String := 'F900 High signal noise detected';
   		        16778239:
   		            qActual_Diagnostics_String := 'F902 Min signal noise detected';
   		        16778242:
   		            qActual_Diagnostics_String := 'F101 Sensor temperature';
   		        16778253:
   		            qActual_Diagnostics_String := 'F062 Sensor connection faulty';
   		        16778254:
   		            qActual_Diagnostics_String := 'F062 Sensor connection faulty';
   		        16778256:
   		            qActual_Diagnostics_String := 'F062 Sensor connection faulty';
   		        16778279:
   		            qActual_Diagnostics_String := 'F806 Loop diagnostics';
   		        16778295:
   		            qActual_Diagnostics_String := 'F272 Main electronics faulty';
   		        16778490:
   		            qActual_Diagnostics_String := 'F419 Power cycle required';
   		        25165849:
   		            qActual_Diagnostics_String := 'F841 Operating range';
   		        25165853:
   		            qActual_Diagnostics_String := 'F081 Sensor initialization faulty';
   		        25165854:
   		            qActual_Diagnostics_String := 'F100 Sensor error';
   		        25165858:
   		            qActual_Diagnostics_String := 'F062 Sensor connection faulty';
   		        25165861:
   		            qActual_Diagnostics_String := 'F822 Sensor temperature out of range';
   		        25165867:
   		            qActual_Diagnostics_String := 'F801 Supply voltage too low';
   		        25165875:
   		            qActual_Diagnostics_String := 'F435 Linearization faulty';
   		        25165891:
   		            qActual_Diagnostics_String := 'F803 Loop current faulty';
   		        25165905:
   		            qActual_Diagnostics_String := 'F102 Sensor incompatible error';
   		        25165920:
   		            qActual_Diagnostics_String := 'F437 Configuration incompatible';
   		        25165922:
   		            qActual_Diagnostics_String := 'F282 Data storage inconsistent';
   		        25165927:
   		            qActual_Diagnostics_String := 'F242 Firmware incompatible';
   		        25165931:
   		            qActual_Diagnostics_String := 'F252 Module incompatible';
   		        25165944:
   		            qActual_Diagnostics_String := 'F270 Main electronics defective';
   		        25165945:
   		            qActual_Diagnostics_String := 'F272 Main electronics faulty';
   		        25165948:
   		            qActual_Diagnostics_String := 'F270 Main electronics defective';
   		        25165949:
   		            qActual_Diagnostics_String := 'F272 Main electronics faulty';
   		        25165951:
   		            qActual_Diagnostics_String := 'F270 Main electronics defective';
   		        25165952:
   		            qActual_Diagnostics_String := 'F270 Main electronics defective';
   		        25165956:
   		            qActual_Diagnostics_String := 'F270 Main electronics defective';
   		        25165963:
   		            qActual_Diagnostics_String := 'F410 Data transfer failed';
   		        25165982:
   		            qActual_Diagnostics_String := 'F283 Memory content inconsistent';
   		        25165983:
   		            qActual_Diagnostics_String := 'F270 Main electronics defective';
   		        25165995:
   		            qActual_Diagnostics_String := 'F270 Main electronics defective';
   		        25165997:
   		            qActual_Diagnostics_String := 'F805 Loop current faulty';
   		        25166049:
   		            qActual_Diagnostics_String := 'F283 Memory content inconsistent';
   		        25166053:
   		            qActual_Diagnostics_String := 'F273 Main electronics defective';
   		        25166054:
   		            qActual_Diagnostics_String := 'F388 Electronics and HistoROM defective';
   		        25166424:
   		            qActual_Diagnostics_String := 'F272 Main electronics faulty';
   		        25166809:
   		            qActual_Diagnostics_String := 'F501 Process alert scaled variable';
   		        25166810:
   		            qActual_Diagnostics_String := 'F906 Out of range signal detected';
   		        25166811:
   		            qActual_Diagnostics_String := 'F500 Process alert pressure';
   		        25166812:
   		            qActual_Diagnostics_String := 'F502 Process alert temperature';
   		        25166845:
   		            qActual_Diagnostics_String := 'F901 Low signal noise detected';
   		        25166846:
   		            qActual_Diagnostics_String := 'F900 High signal noise detected';
   		        25166847:
   		            qActual_Diagnostics_String := 'F902 Min signal noise detected';
   		        25166850:
   		            qActual_Diagnostics_String := 'F101 Sensor temperature';
   		        25166861:
   		            qActual_Diagnostics_String := 'F062 Sensor connection faulty';
   		        25166862:
   		            qActual_Diagnostics_String := 'F062 Sensor connection faulty';
   		        25166864:
   		            qActual_Diagnostics_String := 'F062 Sensor connection faulty';
   		        25166887:
   		            qActual_Diagnostics_String := 'F806 Loop diagnostics';
   		        25166903:
   		            qActual_Diagnostics_String := 'F272 Main electronics faulty';
   		        25167098:
   		            qActual_Diagnostics_String := 'F419 Power cycle required';
   		        33554445:
   		            qActual_Diagnostics_String := 'C485 Process variable simulation active';
   		        33554446:
   		            qActual_Diagnostics_String := 'C491 Current output simulation active';
   		        33554457:
   		            qActual_Diagnostics_String := 'C841 Operating range';
   		        33554469:
   		            qActual_Diagnostics_String := 'C822 Sensor temperature out of range';
   		        33554575:
   		            qActual_Diagnostics_String := 'C494 Switch output simulation active';
   		        33554576:
   		            qActual_Diagnostics_String := 'C484 Failure mode simulation active';
   		        33554948:
   		            qActual_Diagnostics_String := 'C412 Processing download';
   		        33555417:
   		            qActual_Diagnostics_String := 'C501 Process alert scaled variable';
   		        33555418:
   		            qActual_Diagnostics_String := 'C906 Out of range signal detected';
   		        33555419:
   		            qActual_Diagnostics_String := 'C500 Process alert pressure';
   		        33555420:
   		            qActual_Diagnostics_String := 'C502 Process alert temperature';
   		        33555453:
   		            qActual_Diagnostics_String := 'C901 Low signal noise detected';
   		        33555454:
   		            qActual_Diagnostics_String := 'C900 High signal noise detected';
   		        33555455:
   		            qActual_Diagnostics_String := 'C902 Min signal noise detected';
   		        33555495:
   		            qActual_Diagnostics_String := 'C806 Loop diagnostics';
   		        41943053:
   		            qActual_Diagnostics_String := 'C485 Process variable simulation active';
   		        41943054:
   		            qActual_Diagnostics_String := 'C491 Current output simulation active';
   		        41943065:
   		            qActual_Diagnostics_String := 'C841 Operating range';
   		        41943077:
   		            qActual_Diagnostics_String := 'C822 Sensor temperature out of range';
   		        41943183:
   		            qActual_Diagnostics_String := 'C494 Switch output simulation active';
   		        41943184:
   		            qActual_Diagnostics_String := 'C484 Failure mode simulation active';
   		        41943556:
   		            qActual_Diagnostics_String := 'C412 Processing download';
   		        41944025:
   		            qActual_Diagnostics_String := 'C501 Process alert scaled variable';
   		        41944026:
   		            qActual_Diagnostics_String := 'C906 Out of range signal detected';
   		        41944027:
   		            qActual_Diagnostics_String := 'C500 Process alert pressure';
   		        41944028:
   		            qActual_Diagnostics_String := 'C502 Process alert temperature';
   		        41944061:
   		            qActual_Diagnostics_String := 'C901 Low signal noise detected';
   		        41944062:
   		            qActual_Diagnostics_String := 'C900 High signal noise detected';
   		        41944063:
   		            qActual_Diagnostics_String := 'C902 Min signal noise detected';
   		        41944103:
   		            qActual_Diagnostics_String := 'C806 Loop diagnostics';
   		        67108868:
   		            qActual_Diagnostics_String := 'M431 Trim required';
   		        67108889:
   		            qActual_Diagnostics_String := 'M841 Operating range';
   		        67108901:
   		            qActual_Diagnostics_String := 'M822 Sensor temperature out of range';
   		        67108970:
   		            qActual_Diagnostics_String := 'M438 Dataset different';
   		        67109090:
   		            qActual_Diagnostics_String := 'M287 Memory content inconsistent';
   		        67109849:
   		            qActual_Diagnostics_String := 'M501 Process alert scaled variable';
   		        67109850:
   		            qActual_Diagnostics_String := 'M906 Out of range signal detected';
   		        67109851:
   		            qActual_Diagnostics_String := 'M500 Process alert pressure';
   		        67109852:
   		            qActual_Diagnostics_String := 'M502 Process alert temperature';
   		        67109862:
   		            qActual_Diagnostics_String := 'M263 Incompatibility detected';
   		        67109885:
   		            qActual_Diagnostics_String := 'M901 Low signal noise detected';
   		        67109886:
   		            qActual_Diagnostics_String := 'M900 High signal noise detected';
   		        67109887:
   		            qActual_Diagnostics_String := 'M902 Min signal noise detected';
   		        67109896:
   		            qActual_Diagnostics_String := 'M807 No Baseline due to insuf. volt. at 20 mA';
   		        67109927:
   		            qActual_Diagnostics_String := 'M806 Loop diagnostics';
   		        67109944:
   		            qActual_Diagnostics_String := 'M287 Memory content inconsistent';
   		        67110032:
   		            qActual_Diagnostics_String := 'M503 Zero adjustment';
   		        75497476:
   		            qActual_Diagnostics_String := 'M431 Trim required';
   		        75497497:
   		            qActual_Diagnostics_String := 'M841 Operating range';
   		        75497509:
   		            qActual_Diagnostics_String := 'M822 Sensor temperature out of range';
   		        75497578:
   		            qActual_Diagnostics_String := 'M438 Dataset different';
   		        75497698:
   		            qActual_Diagnostics_String := 'M287 Memory content inconsistent';
   		        75498457:
   		            qActual_Diagnostics_String := 'M501 Process alert scaled variable';
   		        75498458:
   		            qActual_Diagnostics_String := 'M906 Out of range signal detected';
   		        75498459:
   		            qActual_Diagnostics_String := 'M500 Process alert pressure';
   		        75498460:
   		            qActual_Diagnostics_String := 'M502 Process alert temperature';
   		        75498470:
   		            qActual_Diagnostics_String := 'M263 Incompatibility detected';
   		        75498493:
   		            qActual_Diagnostics_String := 'M901 Low signal noise detected';
   		        75498494:
   		            qActual_Diagnostics_String := 'M900 High signal noise detected';
   		        75498495:
   		            qActual_Diagnostics_String := 'M902 Min signal noise detected';
   		        75498504:
   		            qActual_Diagnostics_String := 'M807 No Baseline due to insuf. volt. at 20 mA';
   		        75498535:
   		            qActual_Diagnostics_String := 'M806 Loop diagnostics';
   		        75498552:
   		            qActual_Diagnostics_String := 'M287 Memory content inconsistent';
   		        75498640:
   		            qActual_Diagnostics_String := 'M503 Zero adjustment';
   		        134217753:
   		            qActual_Diagnostics_String := 'S841 Operating range';
   		        134217765:
   		            qActual_Diagnostics_String := 'S822 Sensor temperature out of range';
   		        134217772:
   		            qActual_Diagnostics_String := 'S802 Supply voltage too high';
   		        134217863:
   		            qActual_Diagnostics_String := 'S825 Electronics temperature';
   		        134217881:
   		            qActual_Diagnostics_String := 'S441 Current output saturated';
   		        134218639:
   		            qActual_Diagnostics_String := 'S804 Switch output overloaded';
   		        134218713:
   		            qActual_Diagnostics_String := 'S501 Process alert scaled variable';
   		        134218714:
   		            qActual_Diagnostics_String := 'S906 Out of range signal detected';
   		        134218715:
   		            qActual_Diagnostics_String := 'S500 Process alert pressure';
   		        134218716:
   		            qActual_Diagnostics_String := 'S502 Process alert temperature';
   		        134218749:
   		            qActual_Diagnostics_String := 'S901 Low signal noise detected';
   		        134218750:
   		            qActual_Diagnostics_String := 'S900 High signal noise detected';
   		        134218751:
   		            qActual_Diagnostics_String := 'S902 Min signal noise detected';
   		        134218791:
   		            qActual_Diagnostics_String := 'S806 Loop diagnostics';
   		        142606361:
   		            qActual_Diagnostics_String := 'S841 Operating range';
   		        142606373:
   		            qActual_Diagnostics_String := 'S822 Sensor temperature out of range';
   		        142606380:
   		            qActual_Diagnostics_String := 'S802 Supply voltage too high';
   		        142606471:
   		            qActual_Diagnostics_String := 'S825 Electronics temperature';
   		        142606489:
   		            qActual_Diagnostics_String := 'S441 Current output saturated';
   		        142607247:
   		            qActual_Diagnostics_String := 'S804 Switch output overloaded';
   		        142607321:
   		            qActual_Diagnostics_String := 'S501 Process alert scaled variable';
   		        142607322:
   		            qActual_Diagnostics_String := 'S906 Out of range signal detected';
   		        142607323:
   		            qActual_Diagnostics_String := 'S500 Process alert pressure';
   		        142607324:
   		            qActual_Diagnostics_String := 'S502 Process alert temperature';
   		        142607357:
   		            qActual_Diagnostics_String := 'S901 Low signal noise detected';
   		        142607358:
   		            qActual_Diagnostics_String := 'S900 High signal noise detected';
   		        142607359:
   		            qActual_Diagnostics_String := 'S902 Min signal noise detected';
   		        142607399:
   		            qActual_Diagnostics_String := 'S806 Loop diagnostics';
   		        536870937:
   		            qActual_Diagnostics_String := '841 Operating range';
   		        536870949:
   		            qActual_Diagnostics_String := '822 Sensor temperature out of range';
   		        536871262:
   		            qActual_Diagnostics_String := '495 Diagnostic event simulation active';
   		        536871897:
   		            qActual_Diagnostics_String := '501 Process alert scaled variable';
   		        536871898:
   		            qActual_Diagnostics_String := '906 Out of range signal detected';
   		        536871899:
   		            qActual_Diagnostics_String := '500 Process alert pressure';
   		        536871900:
   		            qActual_Diagnostics_String := '502 Process alert temperature';
   		        536871933:
   		            qActual_Diagnostics_String := '901 Low signal noise detected';
   		        536871934:
   		            qActual_Diagnostics_String := '900 High signal noise detected';
   		        536871935:
   		            qActual_Diagnostics_String := '902 Min signal noise detected';
   		        536871975:
   		            qActual_Diagnostics_String := '806 Loop diagnostics';
   		        545259545:
   		            qActual_Diagnostics_String := '841 Operating range';
   		        545259557:
   		            qActual_Diagnostics_String := '822 Sensor temperature out of range';
   		        545259870:
   		            qActual_Diagnostics_String := '495 Diagnostic event simulation active';
   		        545260505:
   		            qActual_Diagnostics_String := '501 Process alert scaled variable';
   		        545260506:
   		            qActual_Diagnostics_String := '906 Out of range signal detected';
   		        545260507:
   		            qActual_Diagnostics_String := '500 Process alert pressure';
   		        545260508:
   		            qActual_Diagnostics_String := '502 Process alert temperature';
   		        545260541:
   		            qActual_Diagnostics_String := '901 Low signal noise detected';
   		        545260542:
   		            qActual_Diagnostics_String := '900 High signal noise detected';
   		        545260543:
   		            qActual_Diagnostics_String := '902 Min signal noise detected';
   		        545260583:
   		            qActual_Diagnostics_String := '806 Loop diagnostics';
   
   					else
   						qActual_Diagnostics_String := 'Error Code unknown';
   
   				end_case;
   
   				Trigger := FALSE;
   				DeviceData.OldState := DeviceData.State;
   		        DeviceData.State := DeviceData.State + 1;
   				DeviceData.CommSuccess := FALSE;
   				DeviceData.AcyclicData[0] := 0;
   				DeviceData.NewState := TRUE;
   
   			 elsif DeviceData.CommTimeOut then
   
   				temp_string1 := 'Error in step ';
   				Temp_DINT := DeviceData.State;
   				DTOS(Temp_DINT, temp_string2);
   				CONCAT(temp_string1, temp_string2, qAOI_Diagnostic_String);
   
   				DeviceData.OldState := DeviceData.State;
   				DeviceData.State := DeviceData.MaxState;
   				DeviceData.CommTimeOut := FALSE;
   				DeviceData.AcyclicData[0] := 0;
   				DeviceData.NewState := TRUE;
   
   		    end_if;
   
   		//*********************************
   	    91: // Last Diagnostic
   	    //*********************************
   
   		    CMD_Index := 298;
   			CMD_Subindex := 0;
   		    CMD_Wr := FALSE;
   			CMD_Rd := TRUE;
   			CMD_ByteLength := 4;
   			Trigger := TRUE;
   
   			if DeviceData.NewState then
   				DeviceData.StateDone := TRUE;
   			end_if;
   
   			if  DeviceData.CommSuccess and DeviceData.ReplayIndex = CMD_Index then
   
   				qLast_Diagnostics_Code	:= DeviceData.AcyclicData[0];
   
   				case qLast_Diagnostics_Code of
   					0:
   	            		qLast_Diagnostics_String := '--------';
   			        16777241:
   			            qLast_Diagnostics_String := 'F841 Operating range';
   			        16777245:
   			            qLast_Diagnostics_String := 'F081 Sensor initialization faulty';
   			        16777246:
   			            qLast_Diagnostics_String := 'F100 Sensor error';
   			        16777250:
   			            qLast_Diagnostics_String := 'F062 Sensor connection faulty';
   			        16777253:
   			            qLast_Diagnostics_String := 'F822 Sensor temperature out of range';
   			        16777259:
   			            qLast_Diagnostics_String := 'F801 Supply voltage too low';
   			        16777267:
   			            qLast_Diagnostics_String := 'F435 Linearization faulty';
   			        16777283:
   			            qLast_Diagnostics_String := 'F803 Loop current faulty';
   			        16777297:
   			            qLast_Diagnostics_String := 'F102 Sensor incompatible error';
   			        16777312:
   			            qLast_Diagnostics_String := 'F437 Configuration incompatible';
   			        16777314:
   			            qLast_Diagnostics_String := 'F282 Data storage inconsistent';
   			        16777319:
   			            qLast_Diagnostics_String := 'F242 Firmware incompatible';
   			        16777323:
   			            qLast_Diagnostics_String := 'F252 Module incompatible';
   			        16777336:
   			            qLast_Diagnostics_String := 'F270 Main electronics defective';
   			        16777337:
   			            qLast_Diagnostics_String := 'F272 Main electronics faulty';
   			        16777340:
   			            qLast_Diagnostics_String := 'F270 Main electronics defective';
   			        16777341:
   			            qLast_Diagnostics_String := 'F272 Main electronics faulty';
   			        16777343:
   			            qLast_Diagnostics_String := 'F270 Main electronics defective';
   			        16777344:
   			            qLast_Diagnostics_String := 'F270 Main electronics defective';
   			        16777348:
   			            qLast_Diagnostics_String := 'F270 Main electronics defective';
   			        16777355:
   			            qLast_Diagnostics_String := 'F410 Data transfer failed';
   			        16777374:
   			            qLast_Diagnostics_String := 'F283 Memory content inconsistent';
   			        16777375:
   			            qLast_Diagnostics_String := 'F270 Main electronics defective';
   			        16777387:
   			            qLast_Diagnostics_String := 'F270 Main electronics defective';
   			        16777389:
   			            qLast_Diagnostics_String := 'F805 Loop current faulty';
   			        16777441:
   			            qLast_Diagnostics_String := 'F283 Memory content inconsistent';
   			        16777445:
   			            qLast_Diagnostics_String := 'F273 Main electronics defective';
   			        16777446:
   			            qLast_Diagnostics_String := 'F388 Electronics and HistoROM defective';
   			        16777816:
   			            qLast_Diagnostics_String := 'F272 Main electronics faulty';
   			        16778201:
   			            qLast_Diagnostics_String := 'F501 Process alert scaled variable';
   			        16778202:
   			            qLast_Diagnostics_String := 'F906 Out of range signal detected';
   			        16778203:
   			            qLast_Diagnostics_String := 'F500 Process alert pressure';
   			        16778204:
   			            qLast_Diagnostics_String := 'F502 Process alert temperature';
   			        16778237:
   			            qLast_Diagnostics_String := 'F901 Low signal noise detected';
   			        16778238:
   			            qLast_Diagnostics_String := 'F900 High signal noise detected';
   			        16778239:
   			            qLast_Diagnostics_String := 'F902 Min signal noise detected';
   			        16778242:
   			            qLast_Diagnostics_String := 'F101 Sensor temperature';
   			        16778253:
   			            qLast_Diagnostics_String := 'F062 Sensor connection faulty';
   			        16778254:
   			            qLast_Diagnostics_String := 'F062 Sensor connection faulty';
   			        16778256:
   			            qLast_Diagnostics_String := 'F062 Sensor connection faulty';
   			        16778279:
   			            qLast_Diagnostics_String := 'F806 Loop diagnostics';
   			        16778295:
   			            qLast_Diagnostics_String := 'F272 Main electronics faulty';
   			        16778490:
   			            qLast_Diagnostics_String := 'F419 Power cycle required';
   			        25165849:
   			            qLast_Diagnostics_String := 'F841 Operating range';
   			        25165853:
   			            qLast_Diagnostics_String := 'F081 Sensor initialization faulty';
   			        25165854:
   			            qLast_Diagnostics_String := 'F100 Sensor error';
   			        25165858:
   			            qLast_Diagnostics_String := 'F062 Sensor connection faulty';
   			        25165861:
   			            qLast_Diagnostics_String := 'F822 Sensor temperature out of range';
   			        25165867:
   			            qLast_Diagnostics_String := 'F801 Supply voltage too low';
   			        25165875:
   			            qLast_Diagnostics_String := 'F435 Linearization faulty';
   			        25165891:
   			            qLast_Diagnostics_String := 'F803 Loop current faulty';
   			        25165905:
   			            qLast_Diagnostics_String := 'F102 Sensor incompatible error';
   			        25165920:
   			            qLast_Diagnostics_String := 'F437 Configuration incompatible';
   			        25165922:
   			            qLast_Diagnostics_String := 'F282 Data storage inconsistent';
   			        25165927:
   			            qLast_Diagnostics_String := 'F242 Firmware incompatible';
   			        25165931:
   			            qLast_Diagnostics_String := 'F252 Module incompatible';
   			        25165944:
   			            qLast_Diagnostics_String := 'F270 Main electronics defective';
   			        25165945:
   			            qLast_Diagnostics_String := 'F272 Main electronics faulty';
   			        25165948:
   			            qLast_Diagnostics_String := 'F270 Main electronics defective';
   			        25165949:
   			            qLast_Diagnostics_String := 'F272 Main electronics faulty';
   			        25165951:
   			            qLast_Diagnostics_String := 'F270 Main electronics defective';
   			        25165952:
   			            qLast_Diagnostics_String := 'F270 Main electronics defective';
   			        25165956:
   			            qLast_Diagnostics_String := 'F270 Main electronics defective';
   			        25165963:
   			            qLast_Diagnostics_String := 'F410 Data transfer failed';
   			        25165982:
   			            qLast_Diagnostics_String := 'F283 Memory content inconsistent';
   			        25165983:
   			            qLast_Diagnostics_String := 'F270 Main electronics defective';
   			        25165995:
   			            qLast_Diagnostics_String := 'F270 Main electronics defective';
   			        25165997:
   			            qLast_Diagnostics_String := 'F805 Loop current faulty';
   			        25166049:
   			            qLast_Diagnostics_String := 'F283 Memory content inconsistent';
   			        25166053:
   			            qLast_Diagnostics_String := 'F273 Main electronics defective';
   			        25166054:
   			            qLast_Diagnostics_String := 'F388 Electronics and HistoROM defective';
   			        25166424:
   			            qLast_Diagnostics_String := 'F272 Main electronics faulty';
   			        25166809:
   			            qLast_Diagnostics_String := 'F501 Process alert scaled variable';
   			        25166810:
   			            qLast_Diagnostics_String := 'F906 Out of range signal detected';
   			        25166811:
   			            qLast_Diagnostics_String := 'F500 Process alert pressure';
   			        25166812:
   			            qLast_Diagnostics_String := 'F502 Process alert temperature';
   			        25166845:
   			            qLast_Diagnostics_String := 'F901 Low signal noise detected';
   			        25166846:
   			            qLast_Diagnostics_String := 'F900 High signal noise detected';
   			        25166847:
   			            qLast_Diagnostics_String := 'F902 Min signal noise detected';
   			        25166850:
   			            qLast_Diagnostics_String := 'F101 Sensor temperature';
   			        25166861:
   			            qLast_Diagnostics_String := 'F062 Sensor connection faulty';
   			        25166862:
   			            qLast_Diagnostics_String := 'F062 Sensor connection faulty';
   			        25166864:
   			            qLast_Diagnostics_String := 'F062 Sensor connection faulty';
   			        25166887:
   			            qLast_Diagnostics_String := 'F806 Loop diagnostics';
   			        25166903:
   			            qLast_Diagnostics_String := 'F272 Main electronics faulty';
   			        25167098:
   			            qLast_Diagnostics_String := 'F419 Power cycle required';
   			        33554445:
   			            qLast_Diagnostics_String := 'C485 Process variable simulation active';
   			        33554446:
   			            qLast_Diagnostics_String := 'C491 Current output simulation active';
   			        33554457:
   			            qLast_Diagnostics_String := 'C841 Operating range';
   			        33554469:
   			            qLast_Diagnostics_String := 'C822 Sensor temperature out of range';
   			        33554575:
   			            qLast_Diagnostics_String := 'C494 Switch output simulation active';
   			        33554576:
   			            qLast_Diagnostics_String := 'C484 Failure mode simulation active';
   			        33554948:
   			            qLast_Diagnostics_String := 'C412 Processing download';
   			        33555417:
   			            qLast_Diagnostics_String := 'C501 Process alert scaled variable';
   			        33555418:
   			            qLast_Diagnostics_String := 'C906 Out of range signal detected';
   			        33555419:
   			            qLast_Diagnostics_String := 'C500 Process alert pressure';
   			        33555420:
   			            qLast_Diagnostics_String := 'C502 Process alert temperature';
   			        33555453:
   			            qLast_Diagnostics_String := 'C901 Low signal noise detected';
   			        33555454:
   			            qLast_Diagnostics_String := 'C900 High signal noise detected';
   			        33555455:
   			            qLast_Diagnostics_String := 'C902 Min signal noise detected';
   			        33555495:
   			            qLast_Diagnostics_String := 'C806 Loop diagnostics';
   			        41943053:
   			            qLast_Diagnostics_String := 'C485 Process variable simulation active';
   			        41943054:
   			            qLast_Diagnostics_String := 'C491 Current output simulation active';
   			        41943065:
   			            qLast_Diagnostics_String := 'C841 Operating range';
   			        41943077:
   			            qLast_Diagnostics_String := 'C822 Sensor temperature out of range';
   			        41943183:
   			            qLast_Diagnostics_String := 'C494 Switch output simulation active';
   			        41943184:
   			            qLast_Diagnostics_String := 'C484 Failure mode simulation active';
   			        41943556:
   			            qLast_Diagnostics_String := 'C412 Processing download';
   			        41944025:
   			            qLast_Diagnostics_String := 'C501 Process alert scaled variable';
   			        41944026:
   			            qLast_Diagnostics_String := 'C906 Out of range signal detected';
   			        41944027:
   			            qLast_Diagnostics_String := 'C500 Process alert pressure';
   			        41944028:
   			            qLast_Diagnostics_String := 'C502 Process alert temperature';
   			        41944061:
   			            qLast_Diagnostics_String := 'C901 Low signal noise detected';
   			        41944062:
   			            qLast_Diagnostics_String := 'C900 High signal noise detected';
   			        41944063:
   			            qLast_Diagnostics_String := 'C902 Min signal noise detected';
   			        41944103:
   			            qLast_Diagnostics_String := 'C806 Loop diagnostics';
   			        67108868:
   			            qLast_Diagnostics_String := 'M431 Trim required';
   			        67108889:
   			            qLast_Diagnostics_String := 'M841 Operating range';
   			        67108901:
   			            qLast_Diagnostics_String := 'M822 Sensor temperature out of range';
   			        67108970:
   			            qLast_Diagnostics_String := 'M438 Dataset different';
   			        67109090:
   			            qLast_Diagnostics_String := 'M287 Memory content inconsistent';
   			        67109849:
   			            qLast_Diagnostics_String := 'M501 Process alert scaled variable';
   			        67109850:
   			            qLast_Diagnostics_String := 'M906 Out of range signal detected';
   			        67109851:
   			            qLast_Diagnostics_String := 'M500 Process alert pressure';
   			        67109852:
   			            qLast_Diagnostics_String := 'M502 Process alert temperature';
   			        67109862:
   			            qLast_Diagnostics_String := 'M263 Incompatibility detected';
   			        67109885:
   			            qLast_Diagnostics_String := 'M901 Low signal noise detected';
   			        67109886:
   			            qLast_Diagnostics_String := 'M900 High signal noise detected';
   			        67109887:
   			            qLast_Diagnostics_String := 'M902 Min signal noise detected';
   			        67109896:
   			            qLast_Diagnostics_String := 'M807 No Baseline due to insuf. volt. at 20 mA';
   			        67109927:
   			            qLast_Diagnostics_String := 'M806 Loop diagnostics';
   			        67109944:
   			            qLast_Diagnostics_String := 'M287 Memory content inconsistent';
   			        67110032:
   			            qLast_Diagnostics_String := 'M503 Zero adjustment';
   			        75497476:
   			            qLast_Diagnostics_String := 'M431 Trim required';
   			        75497497:
   			            qLast_Diagnostics_String := 'M841 Operating range';
   			        75497509:
   			            qLast_Diagnostics_String := 'M822 Sensor temperature out of range';
   			        75497578:
   			            qLast_Diagnostics_String := 'M438 Dataset different';
   			        75497698:
   			            qLast_Diagnostics_String := 'M287 Memory content inconsistent';
   			        75498457:
   			            qLast_Diagnostics_String := 'M501 Process alert scaled variable';
   			        75498458:
   			            qLast_Diagnostics_String := 'M906 Out of range signal detected';
   			        75498459:
   			            qLast_Diagnostics_String := 'M500 Process alert pressure';
   			        75498460:
   			            qLast_Diagnostics_String := 'M502 Process alert temperature';
   			        75498470:
   			            qLast_Diagnostics_String := 'M263 Incompatibility detected';
   			        75498493:
   			            qLast_Diagnostics_String := 'M901 Low signal noise detected';
   			        75498494:
   			            qLast_Diagnostics_String := 'M900 High signal noise detected';
   			        75498495:
   			            qLast_Diagnostics_String := 'M902 Min signal noise detected';
   			        75498504:
   			            qLast_Diagnostics_String := 'M807 No Baseline due to insuf. volt. at 20 mA';
   			        75498535:
   			            qLast_Diagnostics_String := 'M806 Loop diagnostics';
   			        75498552:
   			            qLast_Diagnostics_String := 'M287 Memory content inconsistent';
   			        75498640:
   			            qLast_Diagnostics_String := 'M503 Zero adjustment';
   			        134217753:
   			            qLast_Diagnostics_String := 'S841 Operating range';
   			        134217765:
   			            qLast_Diagnostics_String := 'S822 Sensor temperature out of range';
   			        134217772:
   			            qLast_Diagnostics_String := 'S802 Supply voltage too high';
   			        134217863:
   			            qLast_Diagnostics_String := 'S825 Electronics temperature';
   			        134217881:
   			            qLast_Diagnostics_String := 'S441 Current output saturated';
   			        134218639:
   			            qLast_Diagnostics_String := 'S804 Switch output overloaded';
   			        134218713:
   			            qLast_Diagnostics_String := 'S501 Process alert scaled variable';
   			        134218714:
   			            qLast_Diagnostics_String := 'S906 Out of range signal detected';
   			        134218715:
   			            qLast_Diagnostics_String := 'S500 Process alert pressure';
   			        134218716:
   			            qLast_Diagnostics_String := 'S502 Process alert temperature';
   			        134218749:
   			            qLast_Diagnostics_String := 'S901 Low signal noise detected';
   			        134218750:
   			            qLast_Diagnostics_String := 'S900 High signal noise detected';
   			        134218751:
   			            qLast_Diagnostics_String := 'S902 Min signal noise detected';
   			        134218791:
   			            qLast_Diagnostics_String := 'S806 Loop diagnostics';
   			        142606361:
   			            qLast_Diagnostics_String := 'S841 Operating range';
   			        142606373:
   			            qLast_Diagnostics_String := 'S822 Sensor temperature out of range';
   			        142606380:
   			            qLast_Diagnostics_String := 'S802 Supply voltage too high';
   			        142606471:
   			            qLast_Diagnostics_String := 'S825 Electronics temperature';
   			        142606489:
   			            qLast_Diagnostics_String := 'S441 Current output saturated';
   			        142607247:
   			            qLast_Diagnostics_String := 'S804 Switch output overloaded';
   			        142607321:
   			            qLast_Diagnostics_String := 'S501 Process alert scaled variable';
   			        142607322:
   			            qLast_Diagnostics_String := 'S906 Out of range signal detected';
   			        142607323:
   			            qLast_Diagnostics_String := 'S500 Process alert pressure';
   			        142607324:
   			            qLast_Diagnostics_String := 'S502 Process alert temperature';
   			        142607357:
   			            qLast_Diagnostics_String := 'S901 Low signal noise detected';
   			        142607358:
   			            qLast_Diagnostics_String := 'S900 High signal noise detected';
   			        142607359:
   			            qLast_Diagnostics_String := 'S902 Min signal noise detected';
   			        142607399:
   			            qLast_Diagnostics_String := 'S806 Loop diagnostics';
   			        536870937:
   			            qLast_Diagnostics_String := '841 Operating range';
   			        536870949:
   			            qLast_Diagnostics_String := '822 Sensor temperature out of range';
   			        536871262:
   			            qLast_Diagnostics_String := '495 Diagnostic event simulation active';
   			        536871897:
   			            qLast_Diagnostics_String := '501 Process alert scaled variable';
   			        536871898:
   			            qLast_Diagnostics_String := '906 Out of range signal detected';
   			        536871899:
   			            qLast_Diagnostics_String := '500 Process alert pressure';
   			        536871900:
   			            qLast_Diagnostics_String := '502 Process alert temperature';
   			        536871933:
   			            qLast_Diagnostics_String := '901 Low signal noise detected';
   			        536871934:
   			            qLast_Diagnostics_String := '900 High signal noise detected';
   			        536871935:
   			            qLast_Diagnostics_String := '902 Min signal noise detected';
   			        536871975:
   			            qLast_Diagnostics_String := '806 Loop diagnostics';
   			        545259545:
   			            qLast_Diagnostics_String := '841 Operating range';
   			        545259557:
   			            qLast_Diagnostics_String := '822 Sensor temperature out of range';
   			        545259870:
   			            qLast_Diagnostics_String := '495 Diagnostic event simulation active';
   			        545260505:
   			            qLast_Diagnostics_String := '501 Process alert scaled variable';
   			        545260506:
   			            qLast_Diagnostics_String := '906 Out of range signal detected';
   			        545260507:
   			            qLast_Diagnostics_String := '500 Process alert pressure';
   			        545260508:
   			            qLast_Diagnostics_String := '502 Process alert temperature';
   			        545260541:
   			            qLast_Diagnostics_String := '901 Low signal noise detected';
   			        545260542:
   			            qLast_Diagnostics_String := '900 High signal noise detected';
   			        545260543:
   			            qLast_Diagnostics_String := '902 Min signal noise detected';
   			        545260583:
   			            qLast_Diagnostics_String := '806 Loop diagnostics';
   
   					else
   						qLast_Diagnostics_String := 'Error Code unknown';
   
   				end_case;
   
   				Trigger := FALSE;
   				DeviceData.OldState := DeviceData.State;
   		        DeviceData.State := DeviceData.MaxState;
   				DeviceData.CommSuccess := FALSE;
   				DeviceData.AcyclicData[0] := 0;
   				DeviceData.NewState := TRUE;
   
   			 elsif DeviceData.CommTimeOut then
   
   				temp_string1 := 'Error in step ';
   				Temp_DINT := DeviceData.State;
   				DTOS(Temp_DINT, temp_string2);
   				CONCAT(temp_string1, temp_string2, qAOI_Diagnostic_String);
   
   				DeviceData.OldState := DeviceData.State;
   		        DeviceData.State := DeviceData.MaxState;
   				DeviceData.CommTimeOut := FALSE;
   				DeviceData.AcyclicData[0] := 0;
   				DeviceData.NewState := TRUE;
   
   			end_if;
   
   		//*********************************
   		98: // End Step Trigger Guard
   		//*********************************
   
   				DeviceData.State := 0;
   				CommAOIBusy := 0;
   				DeviceAOISendRequest.[DeviceData.DevicePort] := 0;
   				ActiveComPort := 0;
   				ActiveAOI := 0;
   				DataToSend[0] := 0;
   				DataToSend[1] := 0;
   				DataToSend[2] := 0;
   				DataToSend[3] := 0;
   				DataToSend[4] := 0;
   				DataToSend[5] := 0;
    				DataToSend[6] := 0;
   				DataToSend[7] := 0;
    				DataToSend[8] := 0;
   				DataToSend[9] := 0;
   				DeviceData.StateDone := FALSE;
   				Skip := 0;
   				firstTimeDone := FALSE;
   				DeviceData.NewState := FALSE;
   				DeviceData.OldState := 0;
   				ActiveAOI := FALSE;
   
   				if SimActive then
   
   					SimActive := FALSE;
   					SimChanged := FALSE;
   
   				elsif UnitActive then
   
   					UnitActive := FALSE;
   					UnitChanged := FALSE;
   
   				elsif CondStatusActive then
   
   					CondStatusActive := FALSE;
   					CondStatusChanged := FALSE;
   
   				elsif HeartbeatVerificationActive then
   
   					HeartbeatVerificationActive := FALSE;
   					HeartbeatVerificationChanged := FALSE;
   
   				end_if;
   
   		end_case;
   
   	end_if;
   
   	//*************************
   	// Execution Area
   	//*************************
   	if DeviceData.State > StateMin and DeviceData.State < DeviceData.MaxState then
   
   		DataToSend[2] := DeviceData.DevicePort;
   		DataToSend[3] := CMD_Index;
   		DataToSend[4] := CMD_Subindex;
   		DataToSend[5].0 := CMD_Rd;
   		DataToSend[5].1 := CMD_Wr;
   		DataToSend[5].8 := CMD_ByteLength.0;  // Bits for the Length of the Data
   		DataToSend[5].9 := CMD_ByteLength.1;
   		DataToSend[5].10 := CMD_ByteLength.2;
   		DataToSend[5].11 := CMD_ByteLength.3;
   		DataToSend[5].12 := CMD_ByteLength.4;
   		DataToSend[5].13 := CMD_ByteLength.5;
   		DataToSend[5].14 := CMD_ByteLength.6;
   		DataToSend[5].15 := CMD_ByteLength.7;
   		DataToSend[5].7 := Trigger;
   
   		qCommError := CommError;
   
   	end_if;
   
   
   
END_ROUTINE
END_ADD_ON_INSTRUCTION
